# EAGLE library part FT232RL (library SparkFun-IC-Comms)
FT232RL USB UART FT232RL 4th Generation USB UART (USB <-> Serial) Controller. Datasheet SparkFun Products Component (COM-00650) SparkFun RedBot Mainboard (ROB-12097) SparkFun FTDI Basic Breakout - 5V (DEV-09716) SparkFun FTDI Basic Breakout - 3.3V (DEV-09873) Bus Pirate - v3.6a (TOL-12942) SparkFun USB to Serial Breakout - FT232RL (BOB-12731) SparkFun PicoBoard (WIG-11888) SparkFun RFID USB Reader (SEN-09963) LilyPad FTDI Basic Breakout - 5V (DEV-10275) SparkFun Stepoko (ROB-13899)
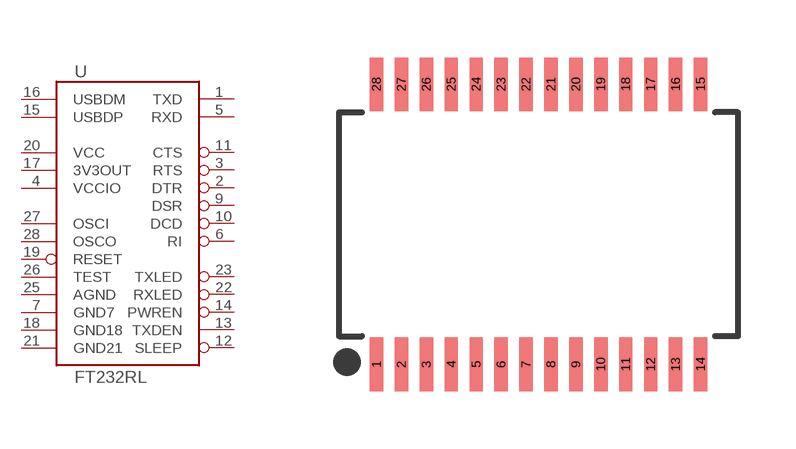
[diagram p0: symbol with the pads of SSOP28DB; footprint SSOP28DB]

Designator prefix U

## FT232RLSSOP (PROD_ID: IC-00870; VALUE: FT232RL)  [SSOP28DB]
1  TXD  out
2  DTR  out
3  RTS  out
4  VCCIO  pwr
5  RXD  in
6  RI  in
7  GND7  pwr
9  DSR  in
10  DCD  in
11  CTS  in
12  SLEEP  in
13  TXDEN  in
14  PWREN  in
15  USBDP
16  USBDM
17  3V3OUT  out
18  GND18  pwr
19  RESET  in
20  VCC  pwr
21  GND21  pwr
22  RXLED  in
23  TXLED  in
25  AGND  pwr
26  TEST  in
27  OSCI  in
28  OSCO  out

## Footprint SSOP28DB (pad centres in mm)
Small Shrink Outline Package - 28 DB Specifications: Pin count: 28 Example device(s): FT232RL
smd 0.348 x 1.397: 1 -4.225,-3.656; 2 -3.575,-3.656; 3 -2.925,-3.656; 4 -2.275,-3.656; 5 -1.625,-3.656; 6 -0.975,-3.656; 7 -0.325,-3.656; 8 0.325,-3.656; 9 0.975,-3.656; 10 1.625,-3.656; 11 2.275,-3.656; 12 2.925,-3.656; 13 3.575,-3.656; 14 4.225,-3.656; 15 4.225,3.656; 16 3.575,3.656; 17 2.925,3.656; 18 2.275,3.656; 19 1.625,3.656; 20 0.975,3.656; 21 0.325,3.656; 22 -0.325,3.656; 23 -0.975,3.656; 24 -1.625,3.656; 25 -2.275,3.656; 26 -2.925,3.656; 27 -3.575,3.656; 28 -4.225,3.656

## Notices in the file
Licensing: Creative Commons ShareAlike 4.0 International - https://creativecommons.org/licenses/by-sa/4.0
